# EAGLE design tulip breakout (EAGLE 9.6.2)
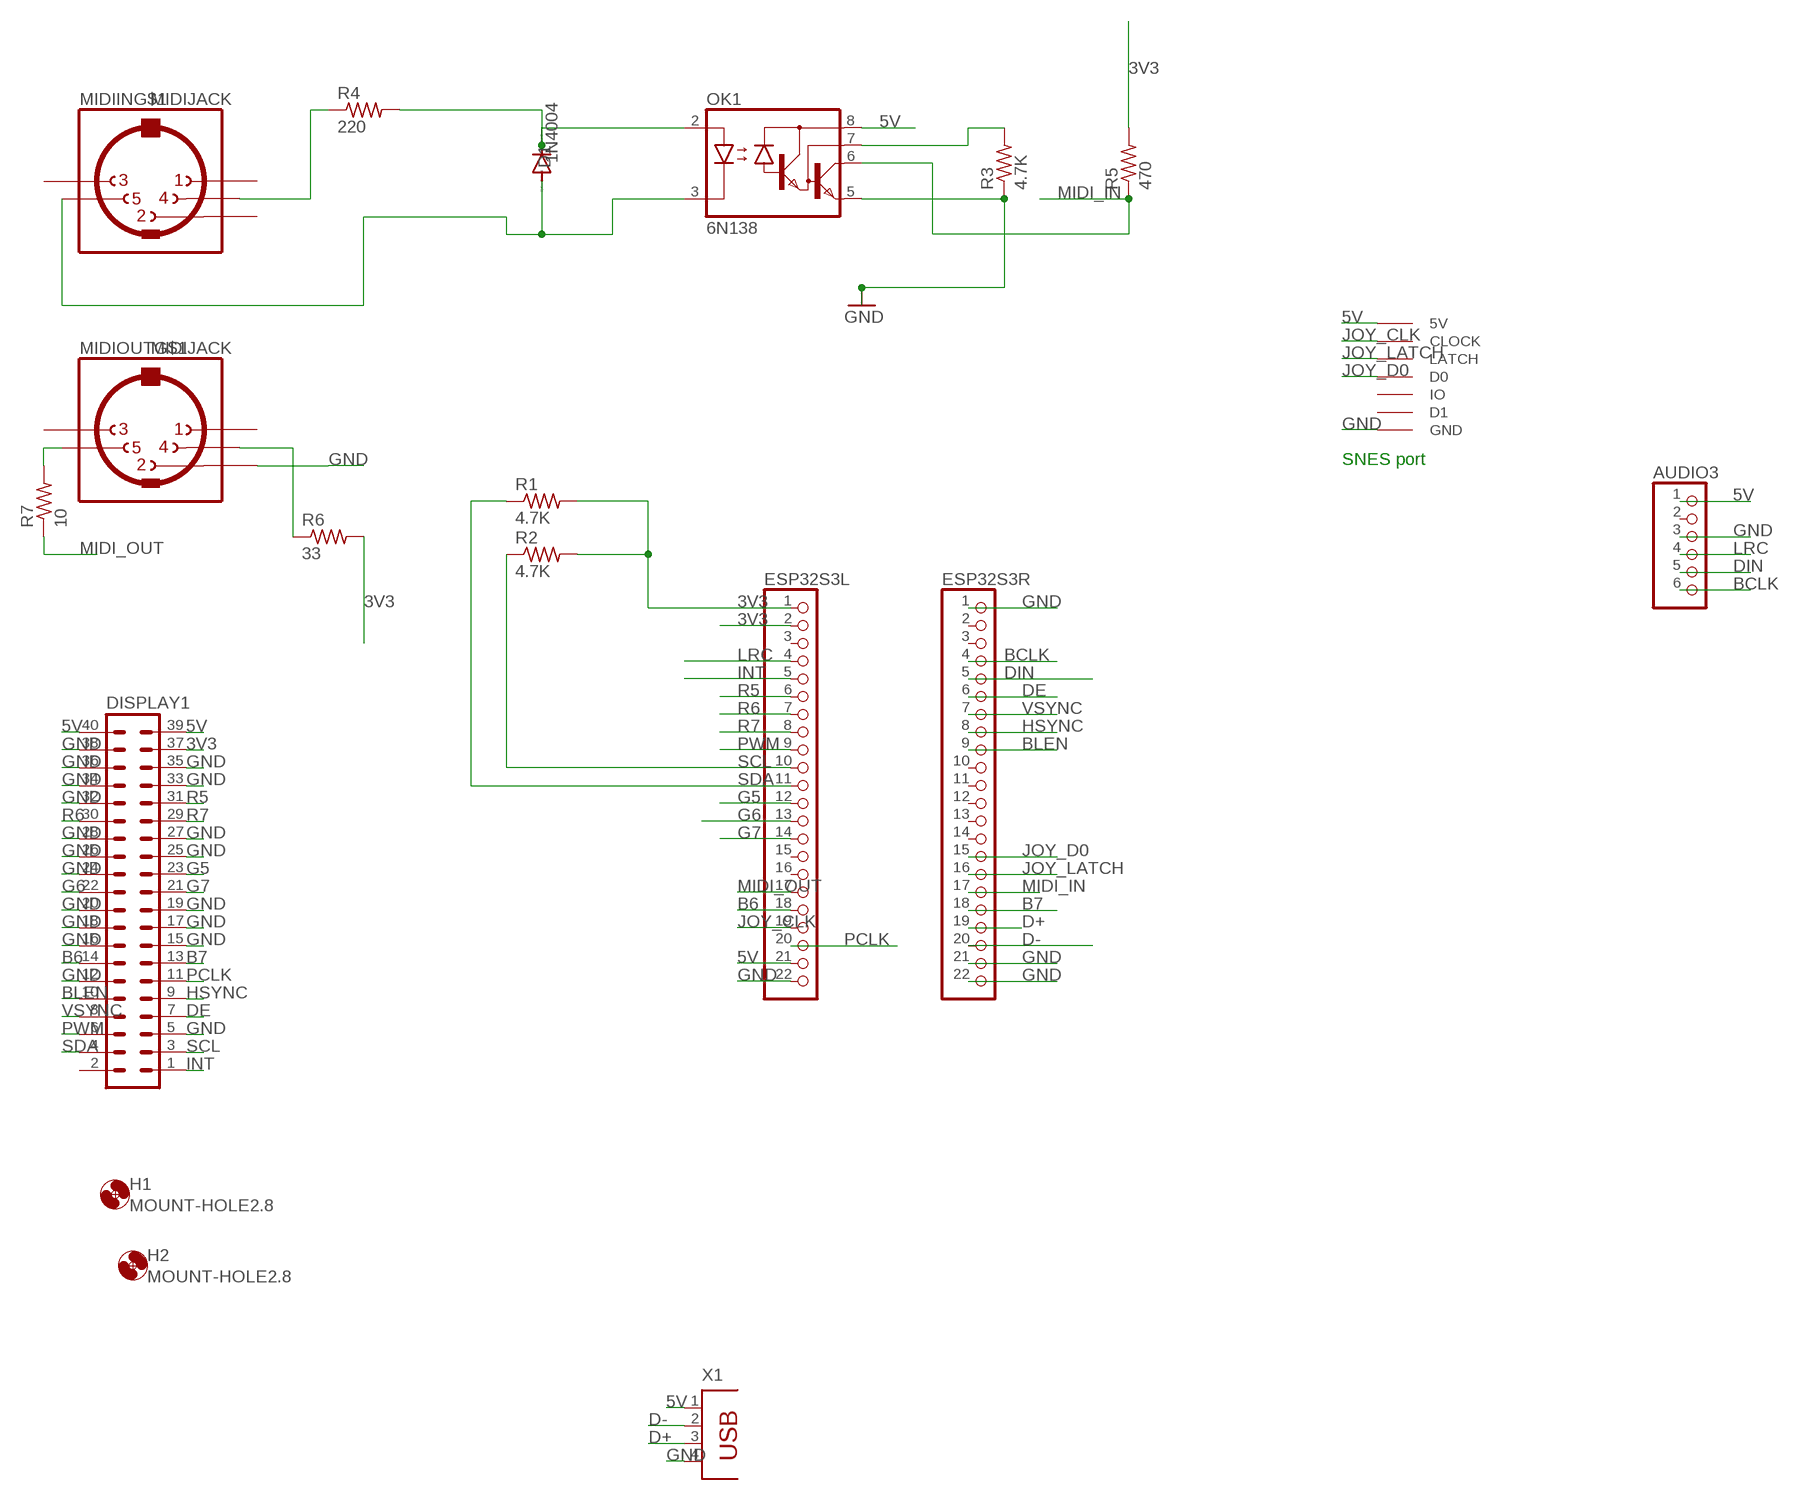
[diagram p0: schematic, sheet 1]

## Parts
AUDIO3  PINHD-1X6  [1X06]
D1  1N4004  [DO41-10]
DISPLAY1  MA20-2  [MA20-2]
ESP32S3L  PINHD-1X22  [1X22]
ESP32S3R  PINHD-1X22  [1X22]
H1  MOUNT-HOLE2.8  [2,8]
H2  MOUNT-HOLE2.8  [2,8]
MIDIIN  MIDIJACK  [CP-2350]
MIDIOUT  MIDIJACK  [CP-2350]
OK1  6N138  [DIL08]
R1  4.7K  R-US_0207/12  [0207/12]
R2  4.7K  R-US_0207/12  [0207/12]
R3  4.7K  R-US_0207/12  [0207/12]
R4  220  R-US_0207/12  [0207/12]
R5  470  R-US_0207/12  [0207/12]
R6  33  R-US_0207/12  [0207/12]
R7  10  R-US_0207/12  [0207/12]
U$2  SNESCONN  [SNESCONN]
X1  PN87520  [PN87520]

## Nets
3V3: DISPLAY1.37 ESP32S3L.1 ESP32S3L.2 R1.2 R2.2 R5.2 R6.2
5V: AUDIO3.1 DISPLAY1.39 DISPLAY1.40 ESP32S3L.21 OK1.8(VCC) U$2.5V X1.1
B6: DISPLAY1.14 ESP32S3L.18
B7: DISPLAY1.13 ESP32S3R.18
BCLK: AUDIO3.6 ESP32S3R.4
BLEN: DISPLAY1.10 ESP32S3R.9
D+: ESP32S3R.19 X1.3
D-: ESP32S3R.20 X1.2
DE: DISPLAY1.7 ESP32S3R.6
DIN: AUDIO3.5 ESP32S3R.5
G5: DISPLAY1.23 ESP32S3L.12
G6: DISPLAY1.22 ESP32S3L.13
G7: DISPLAY1.21 ESP32S3L.14
GND: AUDIO3.3 DISPLAY1.5 DISPLAY1.12 DISPLAY1.15 DISPLAY1.16 DISPLAY1.17 DISPLAY1.18 DISPLAY1.19 DISPLAY1.20 DISPLAY1.24 DISPLAY1.25 DISPLAY1.26 DISPLAY1.27 DISPLAY1.28 DISPLAY1.32 DISPLAY1.33 DISPLAY1.34 DISPLAY1.35 DISPLAY1.36 DISPLAY1.38 ESP32S3L.22 ESP32S3R.1 ESP32S3R.21 ESP32S3R.22 MIDIOUT.2 OK1.5(GND) R3.1 U$2.GND X1.4
HSYNC: DISPLAY1.9 ESP32S3R.8
INT: DISPLAY1.1 ESP32S3L.5
JOY_CLK: ESP32S3L.19 U$2.CLOCK
JOY_D0: ESP32S3R.15 U$2.D0
JOY_LATCH: ESP32S3R.16 U$2.LATCH
LRC: AUDIO3.4 ESP32S3L.4
MIDI_IN: ESP32S3R.17 OK1.6(VO) R5.1
MIDI_OUT: ESP32S3L.17 R7.1
N$29: MIDIIN.4 R4.1
N$30: D1.C OK1.2(A) R4.2
N$31: D1.A MIDIIN.5 OK1.3(C)
N$32: OK1.7(VB) R3.2
N$34: MIDIOUT.5 R7.2
N$35: MIDIOUT.4 R6.1
PCLK: DISPLAY1.11 ESP32S3L.20
PWM: DISPLAY1.6 ESP32S3L.9
R5: DISPLAY1.31 ESP32S3L.6
R6: DISPLAY1.30 ESP32S3L.7
R7: DISPLAY1.29 ESP32S3L.8
SCL: DISPLAY1.3 ESP32S3L.10 R2.1
SDA: DISPLAY1.4 ESP32S3L.11 R1.1
VSYNC: DISPLAY1.8 ESP32S3R.7
Unconnected: AUDIO3.2 DISPLAY1.2 ESP32S3L.3 ESP32S3L.15 ESP32S3L.16 ESP32S3R.2 ESP32S3R.3 ESP32S3R.10 ESP32S3R.11 ESP32S3R.12 ESP32S3R.13 ESP32S3R.14 MIDIIN.1 MIDIIN.2 MIDIIN.3 MIDIIN.PE1(MT) MIDIIN.PE2(MT) MIDIIN.PE(MT) MIDIIN.PE@(MT) MIDIOUT.1 MIDIOUT.3 MIDIOUT.PE1(MT) MIDIOUT.PE2(MT) MIDIOUT.PE(MT) MIDIOUT.PE@(MT) U$2.D1 U$2.IO

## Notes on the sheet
- SNES port

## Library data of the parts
AUDIO3 = pinhead:PINHD-1X6: PIN HEADER
D1 = diode:1N4004: DIODE
DISPLAY1 = con-lstb:MA20-2: PIN HEADER; OC_FARNELL: unknown; OC_NEWARK: unknown
ESP32S3L ESP32S3R = pinhead:PINHD-1X22: PIN HEADER
H1 H2 = holes:MOUNT-HOLE: MOUNTING HOLE with drill center marker
MIDIIN MIDIOUT = adafruit:MIDIJACK: DIN 5 jack also known as MIDI jack A modification of conn-hirshman:MAB5SH with two options for the grounding 'teeth'
OK1 = optocoupler:6N138: MOTOROLA OPTO COUPLER; MF: VISHAY/TELEFUNKEN; MPN: 6N138; OC_FARNELL: 9860150; OC_NEWARK: 35K5294
R1-R7 = rcl:R-US_: RESISTOR, American symbol; SPICEPREFIX: R
U$2 = gamepad-conn:SNESCONN
X1 = con-berg:PN87520: BERG USB connector; OC_FARNELL: unknown; OC_NEWARK: unknown

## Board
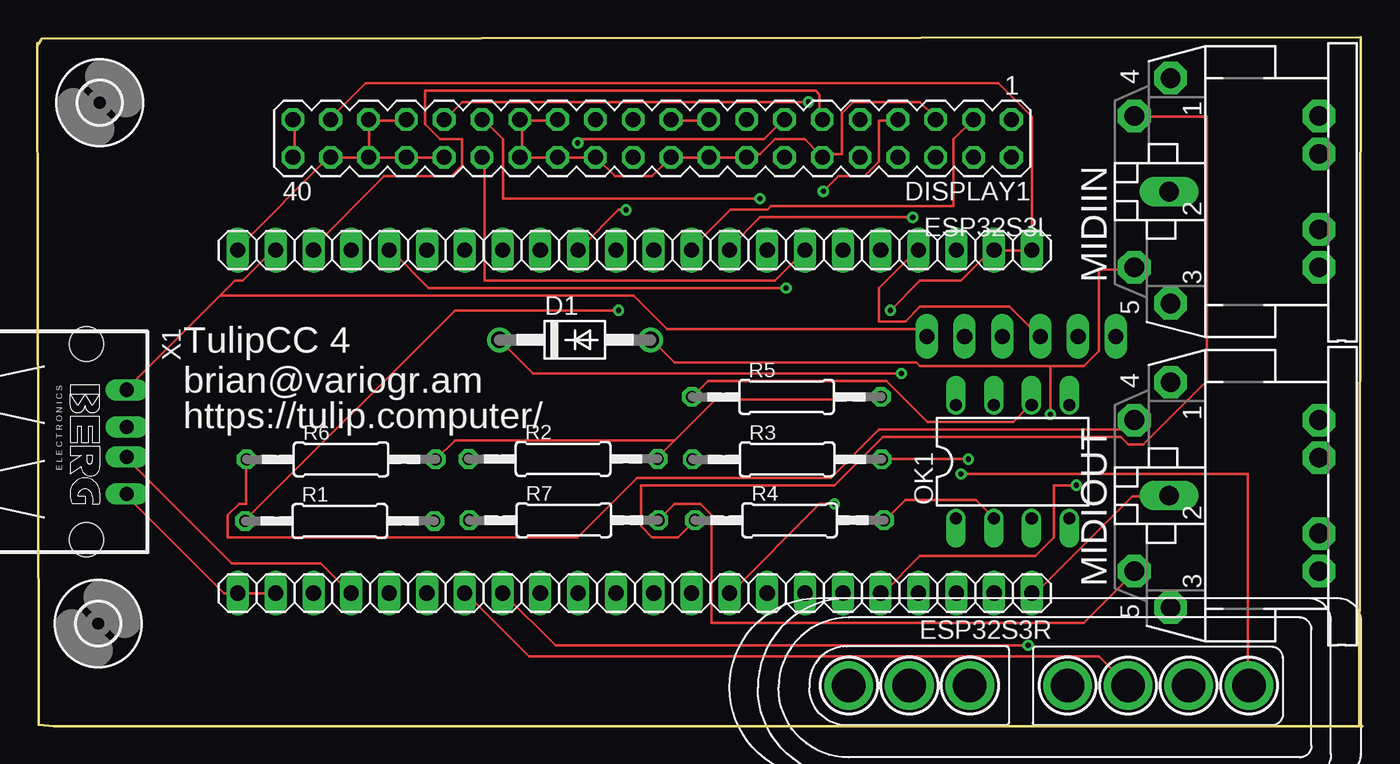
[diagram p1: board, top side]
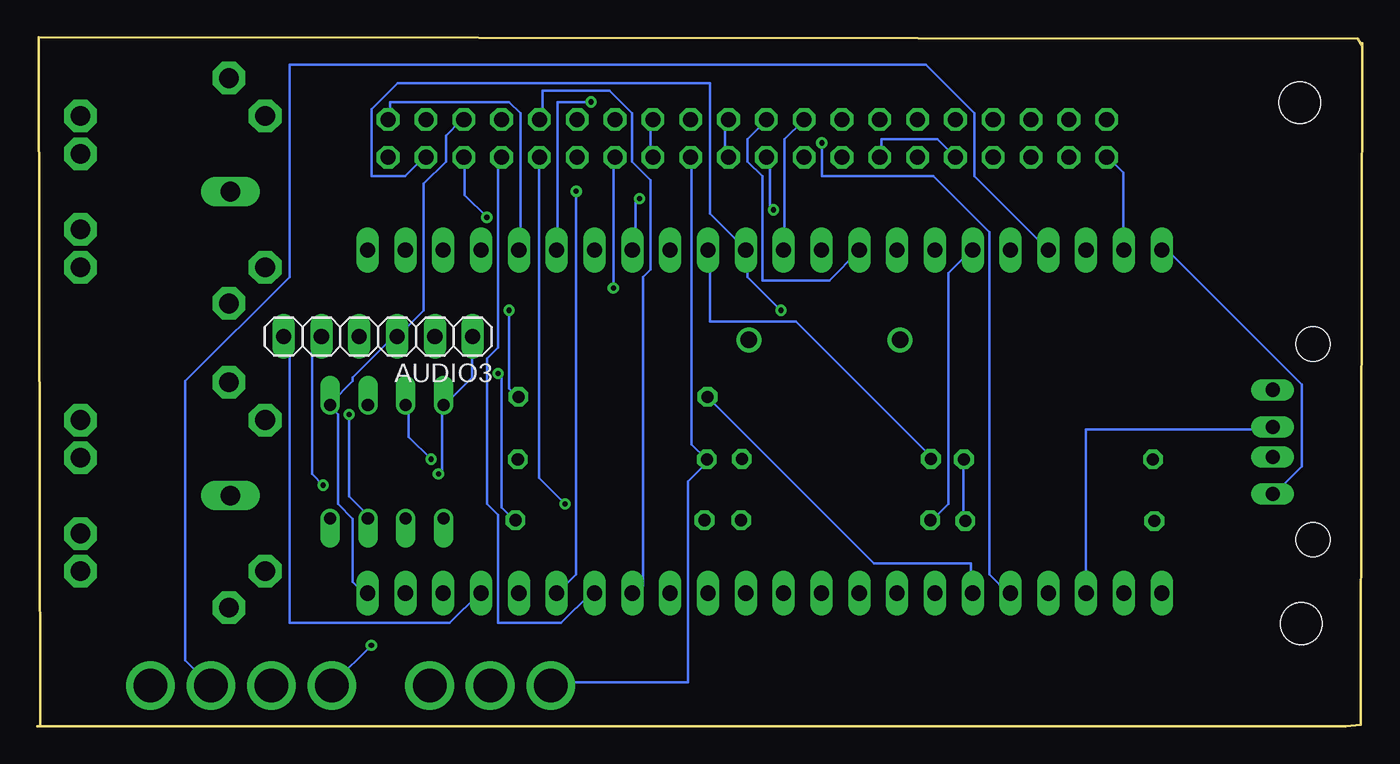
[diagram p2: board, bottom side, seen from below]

Size 89 x 46.3 mm. Coordinates in mm from the lower left corner, seen from the top.
Outline: 0,45.9 0,45.7
Outline: 0,45.7 0.1,2.8
Outline: 88.8,0 88.9,46.3 0.3,46.2 0,45.7
Outline: 89,0 1.1,0 0.1,0.1 0.1,3.3
Copper layers (1*16): Top 0.035mm / dielectric 0.15mm / Bottom 0.035mm
Design rules "default *": minimum track width 6mil, minimum drill 0.35mm, track to track 10mil, track to pad 10mil, pad to pad 10mil, via to via 10mil, smd to smd 10mil, copper to edge 40mil, drill to drill 6mil, minimum pad ring 10mil, minimum via ring 8mil, stop-mask expansion 4mil, vias tented up to drill 0mil, thermal gap 10mil

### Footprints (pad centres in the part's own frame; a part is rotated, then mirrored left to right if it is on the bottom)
1X06 = drill 1.016 long: 1 -6.35,0; 2 -3.81,0; 3 -1.27,0; 4 1.27,0; 5 3.81,0; 6 6.35,0
DO41-10 = drill 1.118: A 5.08,0; C -5.08,0
MA20-2 = drill 1.016 octagon: 1 -24.13,-1.27; 2 -24.13,1.27; 3 -21.59,-1.27; 4 -21.59,1.27; 5 -19.05,-1.27; 6 -19.05,1.27; 7 -16.51,-1.27; 8 -16.51,1.27; 9 -13.97,-1.27; 10 -13.97,1.27; 11 -11.43,-1.27; 12 -11.43,1.27; 13 -8.89,-1.27; 14 -8.89,1.27; 15 -6.35,-1.27; 16 -6.35,1.27; 17 -3.81,-1.27; 18 -3.81,1.27; 19 -1.27,-1.27; 20 -1.27,1.27; 21 1.27,-1.27; 22 1.27,1.27; 23 3.81,-1.27; 24 3.81,1.27; 25 6.35,-1.27; 26 6.35,1.27; 27 8.89,-1.27; 28 8.89,1.27; 29 11.43,-1.27; 30 11.43,1.27; 31 13.97,-1.27; 32 13.97,1.27; 33 16.51,-1.27; 34 16.51,1.27; 35 19.05,-1.27; 36 19.05,1.27; 37 21.59,-1.27; 38 21.59,1.27; 39 24.13,-1.27; 40 24.13,1.27
1X22 = drill 1.016 long: 1 -26.67,0; 2 -24.13,0; 3 -21.59,0; 4 -19.05,0; 5 -16.51,0; 6 -13.97,0; 7 -11.43,0; 8 -8.89,0; 9 -6.35,0; 10 -3.81,0; 11 -1.27,0; 12 1.27,0; 13 3.81,0; 14 6.35,0; 15 8.89,0; 16 11.43,0; 17 13.97,0; 18 16.51,0; 19 19.05,0; 20 21.59,0; 21 24.13,0; 22 26.67,0
2,8 = hole 2.8: 0,0
CP-2350 = drill 1.321 pad 2.184 octagon: 1 7.62,12.58; 3 -7.52,12.58; 4 5.08,15.02; 5 -5.08,15.02; PE -2.54,2.62; PE1 -5.08,2.62; PE2 5.08,2.62; PE@ 2.54,2.62 | drill 1.321 long: 2 0,12.68
DIL08 = drill 0.813 offset: 1 -3.81,-3.81; 2 -1.27,-3.81; 3 1.27,-3.81; 4 3.81,-3.81; 5 3.81,3.81; 6 1.27,3.81; 7 -1.27,3.81; 8 -3.81,3.81
0207/12 = drill 0.813 octagon: 1 -6.35,0; 2 6.35,0
SNESCONN = drill 2.25 pad 3.25: 5V 0,4.064; CLOCK 4.064,4.064; D0 12.192,4.064; D1 18.756,4.064; GND 26.884,4.064; IO 22.82,4.064; LATCH 8.128,4.064
PN87520 = drill 0.95 long: 1 -3.5,2.71; 2 -1,2.71; 3 1,2.71; 4 3.5,2.71 | hole 2.3: -6.57,0; 6.57,0

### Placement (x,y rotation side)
AUDIO3  66.1,26.2 180 bottom
D1  36.12,25.97 0 top
DISPLAY1  41.3,39.5 180 top
ESP32S3L  40.14,32 180 top
ESP32S3R  40.14,8.95 180 top
H1  4.1,6.9 0 top
H2  4.2,41.9 0 top
MIDIIN  88.71,35.93 90 top
MIDIOUT  88.71,15.5 90 top
OK1  65.52,17.78 0 top
R1  20.32,13.79 0 top
R2  35.32,17.97 0 top
R3  50.37,17.94 0 top
R4  50.53,13.85 0 top
R5  50.33,22.14 0 top
R6  20.41,17.94 0 top
R7  35.37,13.85 0 top
U$2  81.4,6.8 180 top
X1  3.31,19.11 270 top

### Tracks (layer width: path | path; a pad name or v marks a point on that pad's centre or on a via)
3V3  (via drill 0.35)
  Top 0.152: 42.8,19.2 45.55,21.95 56.55,21.95 R5.2 | 42.8,19.2 41.8,18.2 R2.2 | 42.8,19.2 28.05,19.2 26.8,17.95 R6.2 | DISPLAY1.37 19.8,40.95 22.05,43.2 64.55,43.2 66.8,40.95 66.8,32.2 ESP32S3L.1 66.8,31.95 64.3,31.95 ESP32S3L.2 64.05,31.95 62.05,29.95 59.3,29.95 v57.3,27.95
  Bottom 0.152: R1.2 26.8,13.95 26.8,17.7 R6.2 | v57.3,27.95 57.3,22.7 56.8,22.2 R5.2
5V  (via drill 0.35)
  Top 0.152: DISPLAY1.40 17.3,38.45 17.3,40.7 DISPLAY1.39 | 12.3,28.95 13.3,29.95 13.8,29.95 15.8,31.95 ESP32S3L.21 | 12.3,28.95 6.05,22.7 X1.1 | 12.3,28.95 40.05,28.95 42.3,26.7 59.05,26.7 59.55,26.2 AUDIO3.1 | v62.05,16.95 81.3,16.95 81.3,2.95 U$2.5V
  Bottom 0.152: AUDIO3.1 59.8,26.2 59.8,23.45 61.55,21.7 OK1.8 61.8,21.45 61.8,17.2 v62.05,16.95 | DISPLAY1.40 17.05,38.2 16.05,37.2 16.05,32.2 ESP32S3L.21
B6  (via drill 0.35)
  Top 0.152: v50.3,29.45 26.3,29.45 23.8,31.95 ESP32S3L.18
  Bottom 0.152: v50.3,29.45 50.3,38.2 DISPLAY1.14
B7  (via drill 0.35)
  Top 0.152: v36.3,39.2 36.55,39.45 48.8,39.45 50.05,40.7 DISPLAY1.13
  Bottom 0.152: v36.3,39.2 36.3,36.95 28.8,36.95 25.05,33.2 25.05,10.2 23.8,8.95 ESP32S3R.18
BCLK
  Bottom 0.152: ESP32S3R.4 59.3,8.95 61.3,6.95 72.05,6.95 72.05,25.95 72.3,26.2 AUDIO3.6
BLEN  (via drill 0.35)
  Top 0.152: v53.55,14.95 52.55,14.95 46.55,8.95 ESP32S3R.9
  Bottom 0.152: v53.55,14.95 55.3,16.7 55.3,38.2 DISPLAY1.10
D+
  Top 0.152: X1.3 6.05,17.95 13.05,10.95 19.05,10.95 21.05,8.95 ESP32S3R.19
D-
  Bottom 0.152: ESP32S3R.20 18.55,19.95 6.05,19.95 X1.2
DE  (via drill 0.35)
  Top 0.152: v52.8,35.95 53.8,36.95 55.55,36.95 56.55,37.95 56.55,40.7 57.8,40.7 DISPLAY1.7
  Bottom 0.152: v52.8,35.95 52.8,10.2 54.05,8.95 ESP32S3R.6
DIN  (via drill 0.35)
  Top 0.152: v69.8,16.2 68.3,16.2 68.3,12.7 67.05,11.45 59.3,11.45 56.8,8.95 ESP32S3R.5
  Bottom 0.152: v69.8,16.2 70.55,16.95 70.55,25.7 70.05,26.2 AUDIO3.5
G5
  Bottom 0.152: ESP32S3L.12 38.8,32.2 38.8,39.45 37.55,40.7 DISPLAY1.23
G6  (via drill 0.35)
  Top 0.152: v39.55,34.7 39.05,34.7 36.55,32.2 ESP32S3L.13
  Bottom 0.152: v39.55,34.7 39.8,34.95 39.8,38.2 DISPLAY1.22
G7
  Bottom 0.152: ESP32S3L.14 33.8,31.95 35.8,29.95 40.3,29.95 40.3,36.95 41.3,37.95 41.3,39.45 40.05,40.7 DISPLAY1.21
GND
  Top 0.152: X1.4 6.05,15.45 12.55,8.95 ESP32S3R.22 ESP32S3R.21 | 22.3,40.7 24.55,40.7 DISPLAY1.33 | DISPLAY1.36 22.3,38.2 24.55,38.2 DISPLAY1.34 24.8,38.2 27.3,38.2 DISPLAY1.32 | 22.3,40.7 22.3,38.45 DISPLAY1.36 | 22.3,40.7 DISPLAY1.35 | ESP32S3L.22 13.55,32.2 19.55,38.2 DISPLAY1.38 19.8,38.2 22.05,38.2 DISPLAY1.36 | ESP32S3R.1 67.05,8.95 73.55,15.45 75.8,15.45 MIDIOUT.2 | 32.55,40.7 34.8,40.7 DISPLAY1.25 | 32.55,40.7 32.55,38.45 DISPLAY1.28 32.55,38.2 34.8,38.2 DISPLAY1.26 35.05,38.2 37.3,38.2 DISPLAY1.24 37.55,38.2 38.8,36.95 41.3,36.95 42.55,38.2 DISPLAY1.20 42.8,38.2 45.05,38.2 DISPLAY1.18 45.3,38.2 47.55,38.2 DISPLAY1.16 47.8,38.45 48.55,38.45 49.55,39.45 51.55,39.45 52.55,38.45 DISPLAY1.12 52.8,38.45 54.05,38.45 54.05,41.2 54.8,41.95 59.3,41.95 60.3,40.95 DISPLAY1.5 | 32.55,40.7 DISPLAY1.27 | DISPLAY1.19 42.8,40.7 45.05,40.7 DISPLAY1.17
  Bottom 0.152: X1.4 5.8,15.7 4.05,17.45 4.05,22.95 13.3,32.2 ESP32S3L.22 | ESP32S3R.1 67.05,8.95 67.8,9.7 67.8,13.95 68.8,14.95 68.8,20.95 69.3,21.45 OK1.5 69.3,21.7 67.8,23.2 67.8,23.45 65.05,26.2 AUDIO3.3 64.8,26.2 63.05,27.95 63.05,36.45 61.55,37.95 61.55,39.7 60.55,40.7 DISPLAY1.5 | DISPLAY1.18 45.05,38.2 45.05,18.95 44.05,17.95 R3.1 44.05,17.7 45.3,16.45 45.3,2.95 54.3,2.95 U$2.GND | DISPLAY1.15 47.8,40.7 47.8,38.45 DISPLAY1.16 | DISPLAY1.19 42.8,40.7 42.8,38.45 DISPLAY1.20 | DISPLAY1.32 28.55,39.45 32.3,39.45 32.3,38.45 DISPLAY1.28
HSYNC
  Bottom 0.152: ESP32S3R.8 48.8,8.95 48.3,9.45 48.3,30.2 47.8,30.7 47.8,36.7 49.05,37.95 49.05,41.2 50.55,42.7 55.05,42.7 55.05,40.95 DISPLAY1.9
INT
  Bottom 0.152: ESP32S3L.5 56.55,32.2 56.55,41.2 57.3,41.95 65.3,41.95 65.3,40.95 DISPLAY1.1
JOY_CLK
  Bottom 0.152: U$2.CLOCK 79.05,4.45 79.05,23.2 72.05,30.2 72.05,44.45 29.3,44.45 26.05,41.2 26.05,36.95 21.3,32.2 ESP32S3L.19
JOY_D0  (via drill 0.35)
  Top 0.152: v66.55,5.45 34.8,5.45 31.3,8.95 ESP32S3R.15
  Bottom 0.152: v66.55,5.45 69.05,2.95 U$2.D0
JOY_LATCH
  Top 0.152: ESP32S3R.16 28.8,8.95 33.05,4.7 71.3,4.7 73.05,2.95 U$2.LATCH
LRC
  Top 0.152: ESP32S3L.4 59.05,31.95 56.55,29.45 56.55,27.2 58.3,27.2 59.3,28.2 65.3,28.2 67.3,26.2 AUDIO3.4
MIDI_IN
  Top 0.152: OK1.6 66.55,21.45 65.55,20.45 59.8,20.45 57.05,23.2 45.05,23.2 44.05,22.2 R5.1
  Bottom 0.152: R5.1 43.8,21.95 32.8,10.95 26.3,10.95 26.3,8.95 ESP32S3R.17
MIDI_OUT
  Bottom 0.152: R7.1 28.8,13.95 27.8,14.95 27.8,30.45 26.3,31.95 ESP32S3L.17
N$29
  Top 0.152: R4.1 44.05,13.7 43.05,12.7 41.3,12.7 40.55,13.45 40.55,16.2 53.55,16.2 56.8,19.45 72.8,19.45 73.3,18.95 74.3,18.95 78.55,23.2 78.55,40.95 73.8,40.95 MIDIIN.4
N$30  (via drill 0.35)
  Top 0.152: R4.2 57.05,13.95 58.3,15.2 63.05,15.2 64.05,14.2 OK1.2 | v58.05,23.7 33.3,23.7 31.05,25.95 D1.C
  Bottom 0.152: v58.05,23.7 57.8,23.45 57.8,14.7 57.05,13.95 R4.2
N$31  (via drill 0.35)
  Top 0.152: 68.05,24.2 v68.05,20.95 | 68.05,24.2 70.3,24.2 71.3,25.2 71.3,30.7 73.55,30.7 MIDIIN.5 | 68.05,24.2 59.3,24.2 59.05,24.45 42.8,24.45 41.3,25.95 D1.A
  Bottom 0.152: v68.05,20.95 68.05,15.45 66.8,14.2 OK1.3
N$32  (via drill 0.35)
  Top 0.152: v62.55,17.95 56.8,17.95 R3.2
  Bottom 0.152: v62.55,17.95 64.05,19.45 64.05,21.45 OK1.7
N$34
  Top 0.152: R7.2 41.8,13.95 42.8,14.95 44.55,14.95 45.3,14.2 45.3,6.95 70.3,6.95 73.55,10.2 MIDIOUT.5
N$35
  Top 0.152: R6.1 14.05,17.7 14.05,14.95 13.55,14.95 12.8,14.2 12.8,12.7 36.3,12.7 40.3,16.7 53.3,16.7 56.55,19.95 73.05,19.95 73.55,20.45 MIDIOUT.4
PCLK
  Top 0.152: ESP32S3L.20 18.55,32.2 23.3,36.95 27.8,36.95 28.55,37.7 28.55,39.45 27.05,39.45 26.05,40.45 26.05,42.7 52.3,42.7 52.55,42.45 52.55,40.95 DISPLAY1.11
PWM  (via drill 0.35)
  Top 0.152: v58.8,34.2 48.55,34.2 46.55,32.2 ESP32S3L.9
  Bottom 0.152: v58.8,34.2 60.3,35.7 60.3,38.2 DISPLAY1.6
R5  (via drill 0.35)
  Top 0.152: v51.8,41.95 28.55,41.95 27.55,40.95 DISPLAY1.31
  Bottom 0.152: v51.8,41.95 54.05,41.95 54.05,32.2 ESP32S3L.6
R6
  Top 0.152: DISPLAY1.30 30.05,38.2 30.05,29.95 49.55,29.95 51.55,31.95 ESP32S3L.7
R7  (via drill 0.35)
  Top 0.152: v48.55,35.45 31.3,35.45 31.3,39.45 30.05,40.7 DISPLAY1.29
  Bottom 0.152: v48.55,35.45 48.8,35.2 48.8,32.2 ESP32S3L.8
SCL
  Top 0.152: DISPLAY1.3 62.8,40.7 61.55,39.45 61.55,34.95 49.3,34.95 49.05,34.7 46.55,34.7 44.05,32.2 ESP32S3L.10
  Bottom 0.152: R2.1 29.05,18.2 38.05,27.2 43.8,27.2 43.8,31.95 ESP32S3L.10
SDA  (via drill 0.35)
  Top 0.152: v39.05,27.95 28.05,27.95 14.05,13.95 R1.1
  Bottom 0.152: v39.05,27.95 41.3,30.2 41.3,31.95 ESP32S3L.11 41.55,32.2 43.8,34.45 43.8,43.2 64.8,43.2 66.55,41.45 66.55,36.95 64.3,36.95 63.05,38.2 DISPLAY1.4
VSYNC
  Bottom 0.152: ESP32S3R.7 51.8,8.95 53.8,6.95 58.05,6.95 58.05,14.2 58.8,14.95 58.8,24.7 58.05,25.45 58.05,38.2 DISPLAY1.8

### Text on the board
tPlace: TulipCC 4 / brian@variogr.am | https://tulip.computer/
